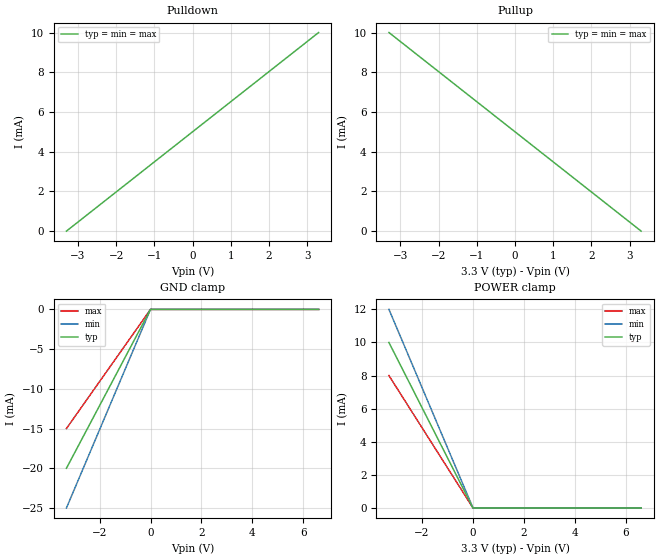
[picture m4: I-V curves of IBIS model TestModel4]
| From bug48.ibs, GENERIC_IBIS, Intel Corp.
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[Model]   TestModel4
Model_type   I/O
Polarity   Non-Inverting
| ... these are OK for an I/O model type
Vinl = 800mV
Vinh = 2.0V
| ... these are OK for an I/O model type
Cref = 10.0pF
Vref = 0.0
Rref = 25
C_comp   5.00pF   4.00pF   6.00pF
[Model Spec]
| ... this is OK for an output model type
| ... and should be used to check the output drive
Vmeas   1.3   1.2   1.5
| ... these should all be OK for an IO model type
Vinl   1   NA   NA
Vinh   1   NA   NA
Vinl+   1   NA   NA
Vinl-   1   NA   NA
Vinh+   1   NA   NA
Vinh-   1   NA   NA
D_overshoot_high   .2   NA   NA
D_overshoot_low   -0.2   NA   NA
S_overshoot_low   -0.1   NA   NA
S_overshoot_high   .1   NA   NA
D_overshoot_time   1n   NA   NA
Pulse_high   3   NA   NA
Pulse_low   0.5   NA   NA
Pulse_time   1n   NA   NA
[Temperature Range]   27.00   100.00   0.00
[Voltage Range]   3.30V   3.00V   3.60V
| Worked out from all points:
|   slope of the pulldown table from 0 to 0.495 V, typ, clamps not added: 660 ohm
|   slope of the pullup table from 0 to 0.495 V, typ, clamps not added: 660 ohm
[GND Clamp]
| voltage   I(typ)   I(min)   I(max)
-3.3V     -20mA      -25mA      -15mA
0V        0A         -5nA       -5nA
3.3V      0A         0A         0A
6.6V      0A         0A         0A
[Power Clamp]
| voltage   I(typ)   I(min)   I(max)
-3.3V     10mA       12mA       8mA
0V        0A         300nA      300nA
3.3V      0A         0A         0A
6.6V      0A         0A         0A
[Pullup]
-3.3V     10mA       10mA       10mA
3.3V      0A         0A         0A
[Pulldown]
-3.3V     0A         0A         0A
3.3V      10mA       10mA       10mA
[Ramp]
dV/dt_r   1.5/.6n NA NA
dV/dt_f   1.5/.6n NA NA
